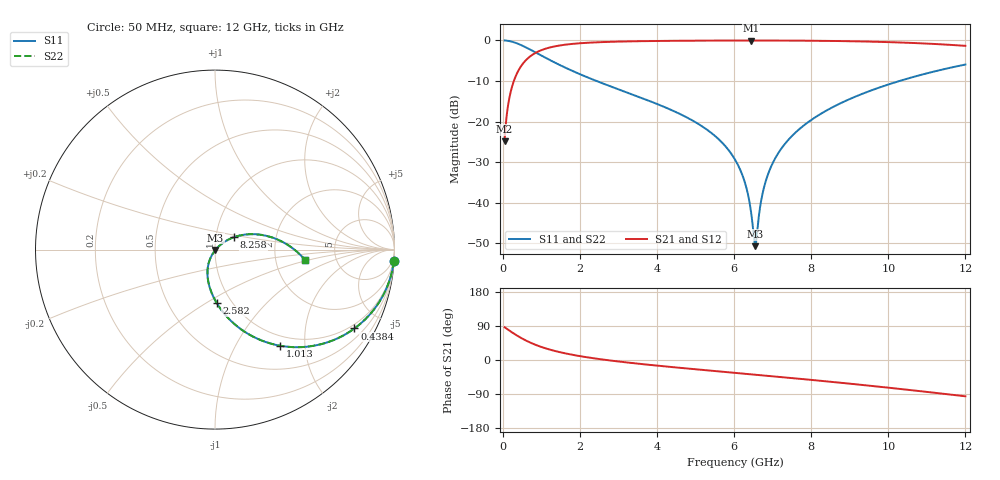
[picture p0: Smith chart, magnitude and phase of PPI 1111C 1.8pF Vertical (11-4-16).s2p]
# GHz S MA R 50
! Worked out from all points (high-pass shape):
!   1601 points, 50 MHz to 12 GHz, reference 50 ohm
!   highest |S21| = -0.03 dB at 6.443 GHz (marker M1); lowest = -24.8 dB at 50 MHz (marker M2)
!   |S21| within 3 dB of the highest: 860.6 MHz to end of sweep
!   lowest |S11| = -50.7 dB at 6.548 GHz (marker M3), VSWR 1.01, Z = 50.2 - j0.196 ohm
!   |S11| at or under -10 dB: 2.434 GHz to 10.29 GHz (7.855 GHz wide, 123 % of centre)
!   |S22| runs from -50.7 to 0.0 dB; largest |S21 - S12| = 0
!   S11 on the Smith chart (normalised r, x): 50 MHz: 1, -32; 438.4 MHz: 0.84, -3.62; 1.013 GHz: 0.84, -1.55; 2.582 GHz: 0.85, -0.55; 8.258 GHz: 1.22, +0.17; 12 GHz: 2.96, -0.45
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0.05  0.9983 -3.6  0.05743 86.4  0.05743 86.4  0.9983 -3.6
0.2068437  0.9728 -14.7  0.2316 75.3  0.2316 75.3  0.9728 -14.7
0.438375  0.8924 -29.5  0.4508 60.5  0.4508 60.5  0.8924 -29.5
1.013469  0.647 -55.9  0.7617 34.1  0.7617 34.1  0.647 -55.9
1.469062  0.5008 -68.9  0.8645 21.0  0.8645 21.0  0.5008 -68.9
2.044156  0.3763 -80.3  0.9251 9.5  0.9251 9.5  0.3763 -80.3
2.581906  0.2969 -88.3  0.9533 1.4  0.9533 1.4  0.2969 -88.3
4.038312  0.1623 -104.5  0.9845 -15.2  0.9845 -15.2  0.1623 -104.5
5.300531  0.07939 -115.5  0.9941 -27.3  0.9941 -27.3  0.07939 -115.5
6.025  0.03407 -119.4  0.9964 -33.9  0.9964 -33.9  0.03407 -119.4
6.286406  0.01746 -117.1  0.9967 -36.3  0.9967 -36.3  0.01746 -117.1
6.44325  0.007598 -105.6  0.9967 -37.8  0.9967 -37.8  0.007598 -105.6
6.510469  0.003909 -80.5  0.9967 -38.4  0.9967 -38.4  0.003909 -80.5
6.547813  0.002921 -41.8  0.9967 -38.7  0.9967 -38.7  0.002921 -41.8
6.592625  0.004065 4.6  0.9967 -39.1  0.9967 -39.1  0.004065 4.6
6.764406  0.01463 37.4  0.9965 -40.7  0.9965 -40.7  0.01463 37.4
6.995938  0.03032 41.2  0.996 -42.9  0.996 -42.9  0.03032 41.2
7.406719  0.05947 40.1  0.9945 -46.8  0.9945 -46.8  0.05947 40.1
8.019156  0.1061 35.4  0.9903 -52.6  0.9903 -52.6  0.1061 35.4
8.258156  0.1253 33.3  0.9879 -55.0  0.9879 -55.0  0.1253 33.3
10.01331  0.2876 15.9  0.9525 -73.1  0.9525 -73.1  0.2876 15.9
12  0.5045 -6.4  0.8568 -95.8  0.8568 -95.8  0.5045 -6.4
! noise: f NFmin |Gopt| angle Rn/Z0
0.05  0.0005986  0.9458  2.788  0.002473
1.372  0.003906  0.689  11  0.00242
2.701  0.006432  0.6403  18.28  0.003296
4.031  0.008742  0.618  25.6  0.004065
5.36  0.011  0.6096  32.69  0.004834
6.682  0.01329  0.6111  39.41  0.005662
8.012  0.01573  0.6202  45.8  0.006619
9.341  0.01837  0.6354  51.82  0.007767
10.67  0.02132  0.6557  57.5  0.009192
12  0.02469  0.6801  62.89  0.01101
